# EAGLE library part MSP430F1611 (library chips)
IC MCU 16BIT 48KB FLASH
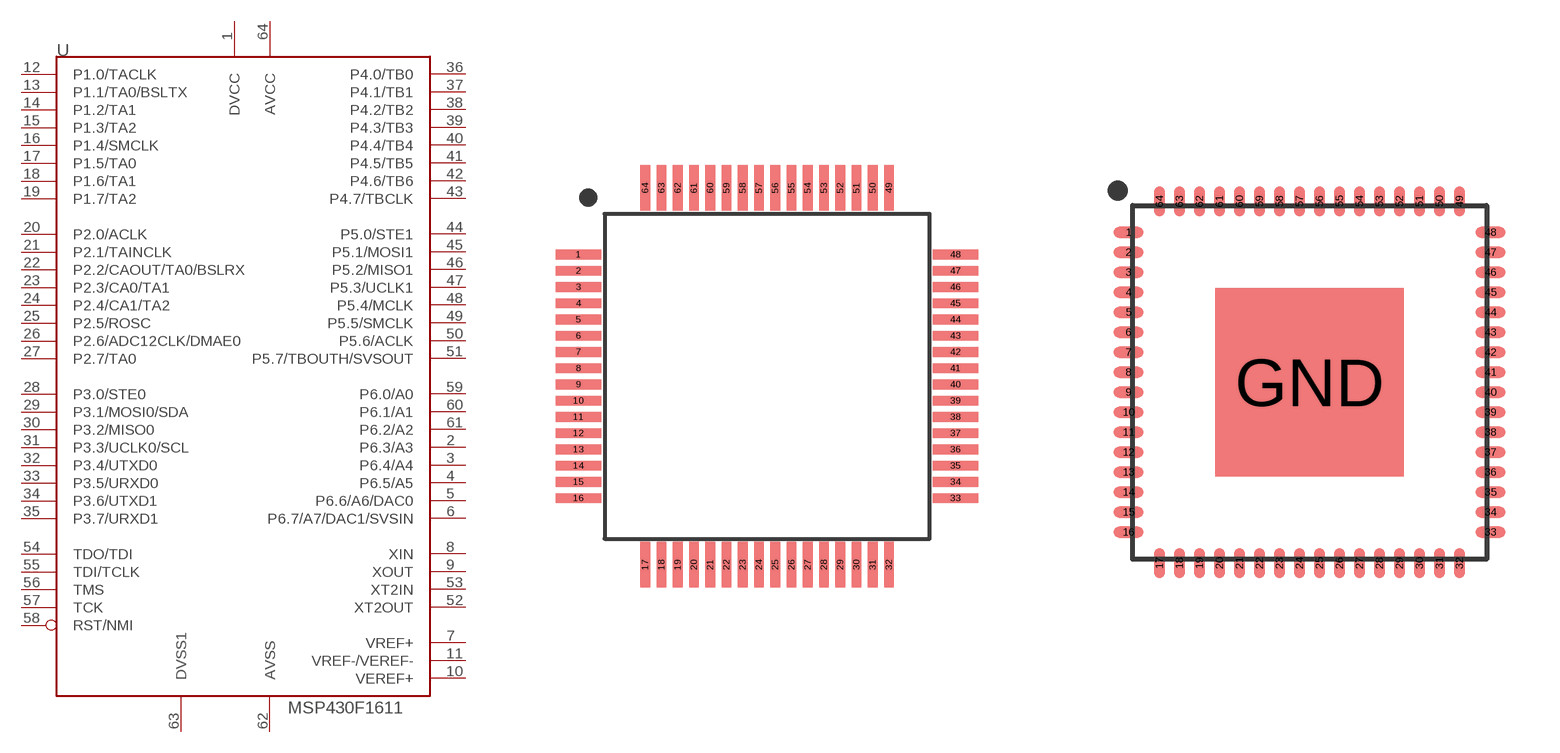
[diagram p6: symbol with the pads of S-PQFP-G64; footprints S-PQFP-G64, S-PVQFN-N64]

Designator prefix U

## MSP430F1611IPM (DIGIKEY: 296-26188-1-ND)  [S-PQFP-G64]
1  DVCC  pwr
2  P6.3/A3
3  P6.4/A4
4  P6.5/A5
5  P6.6/A6/DAC0
6  P6.7/A7/DAC1/SVSIN
7  VREF+
8  XIN
9  XOUT
10  VEREF+
11  VREF-/VEREF-
12  P1.0/TACLK
13  P1.1/TA0/BSLTX
14  P1.2/TA1
15  P1.3/TA2
16  P1.4/SMCLK
17  P1.5/TA0
18  P1.6/TA1
19  P1.7/TA2
20  P2.0/ACLK
21  P2.1/TAINCLK
22  P2.2/CAOUT/TA0/BSLRX
23  P2.3/CA0/TA1
24  P2.4/CA1/TA2
25  P2.5/ROSC
26  P2.6/ADC12CLK/DMAE0
27  P2.7/TA0
28  P3.0/STE0
29  P3.1/MOSI0/SDA
30  P3.2/MISO0
31  P3.3/UCLK0/SCL
32  P3.4/UTXD0
33  P3.5/URXD0
34  P3.6/UTXD1
35  P3.7/URXD1
36  P4.0/TB0
37  P4.1/TB1
38  P4.2/TB2
39  P4.3/TB3
40  P4.4/TB4
41  P4.5/TB5
42  P4.6/TB6
43  P4.7/TBCLK
44  P5.0/STE1
45  P5.1/MOSI1
46  P5.2/MISO1
47  P5.3/UCLK1
48  P5.4/MCLK
49  P5.5/SMCLK
50  P5.6/ACLK
51  P5.7/TBOUTH/SVSOUT
52  XT2OUT
53  XT2IN
54  TDO/TDI
55  TDI/TCLK
56  TMS
57  TCK
58  RST/NMI
59  P6.0/A0
60  P6.1/A1
61  P6.2/A2
62  AVSS  pwr
63  DVSS1  pwr
64  AVCC  pwr

## MSP430F1611IRTD (DIGIKEY: 296-18102-1-ND)  [S-PVQFN-N64]
1  DVCC  pwr
2  P6.3/A3
3  P6.4/A4
4  P6.5/A5
5  P6.6/A6/DAC0
6  P6.7/A7/DAC1/SVSIN
7  VREF+
8  XIN
9  XOUT
10  VEREF+
11  VREF-/VEREF-
12  P1.0/TACLK
13  P1.1/TA0/BSLTX
14  P1.2/TA1
15  P1.3/TA2
16  P1.4/SMCLK
17  P1.5/TA0
18  P1.6/TA1
19  P1.7/TA2
20  P2.0/ACLK
21  P2.1/TAINCLK
22  P2.2/CAOUT/TA0/BSLRX
23  P2.3/CA0/TA1
24  P2.4/CA1/TA2
25  P2.5/ROSC
26  P2.6/ADC12CLK/DMAE0
27  P2.7/TA0
28  P3.0/STE0
29  P3.1/MOSI0/SDA
30  P3.2/MISO0
31  P3.3/UCLK0/SCL
32  P3.4/UTXD0
33  P3.5/URXD0
34  P3.6/UTXD1
35  P3.7/URXD1
36  P4.0/TB0
37  P4.1/TB1
38  P4.2/TB2
39  P4.3/TB3
40  P4.4/TB4
41  P4.5/TB5
42  P4.6/TB6
43  P4.7/TBCLK
44  P5.0/STE1
45  P5.1/MOSI1
46  P5.2/MISO1
47  P5.3/UCLK1
48  P5.4/MCLK
49  P5.5/SMCLK
50  P5.6/ACLK
51  P5.7/TBOUTH/SVSOUT
52  XT2OUT
53  XT2IN
54  TDO/TDI
55  TDI/TCLK
56  TMS
57  TCK
58  RST/NMI
59  P6.0/A0
60  P6.1/A1
61  P6.2/A2
62  AVSS  pwr
63  DVSS1  pwr
64  AVCC  pwr
GND  DVSS1  pwr

## Footprint S-PQFP-G64 (pad centres in mm)
smd 1.4 x 0.3: 1 -5.8,3.75; 2 -5.8,3.25; 3 -5.8,2.75; 4 -5.8,2.25; 5 -5.8,1.75; 6 -5.8,1.25; 7 -5.8,0.75; 8 -5.8,0.25; 9 -5.8,-0.25; 10 -5.8,-0.75; 11 -5.8,-1.25; 12 -5.8,-1.75; 13 -5.8,-2.25; 14 -5.8,-2.75; 15 -5.8,-3.25; 16 -5.8,-3.75; 33 5.8,-3.75; 34 5.8,-3.25; 35 5.8,-2.75; 36 5.8,-2.25; 37 5.8,-1.75; 38 5.8,-1.25; 39 5.8,-0.75; 40 5.8,-0.25; 41 5.8,0.25; 42 5.8,0.75; 43 5.8,1.25; 44 5.8,1.75; 45 5.8,2.25; 46 5.8,2.75; 47 5.8,3.25; 48 5.8,3.75
smd 0.3 x 1.4: 17 -3.75,-5.8; 18 -3.25,-5.8; 19 -2.75,-5.8; 20 -2.25,-5.8; 21 -1.75,-5.8; 22 -1.25,-5.8; 23 -0.75,-5.8; 24 -0.25,-5.8; 25 0.25,-5.8; 26 0.75,-5.8; 27 1.25,-5.8; 28 1.75,-5.8; 29 2.25,-5.8; 30 2.75,-5.8; 31 3.25,-5.8; 32 3.75,-5.8; 49 3.75,5.8; 50 3.25,5.8; 51 2.75,5.8; 52 2.25,5.8; 53 1.75,5.8; 54 1.25,5.8; 55 0.75,5.8; 56 0.25,5.8; 57 -0.25,5.8; 58 -0.75,5.8; 59 -1.25,5.8; 60 -1.75,5.8; 61 -2.25,5.8; 62 -2.75,5.8; 63 -3.25,5.8; 64 -3.75,5.8

## Footprint S-PVQFN-N64 (pad centres in mm)
smd 0.75 x 0.28: 1 -4.525,3.75; 2 -4.525,3.25; 3 -4.525,2.75; 4 -4.525,2.25; 5 -4.525,1.75; 6 -4.525,1.25; 7 -4.525,0.75; 8 -4.525,0.25; 9 -4.525,-0.25; 10 -4.525,-0.75; 11 -4.525,-1.25; 12 -4.525,-1.75; 13 -4.525,-2.25; 14 -4.525,-2.75; 15 -4.525,-3.25; 16 -4.525,-3.75; 33 4.525,-3.75; 34 4.525,-3.25; 35 4.525,-2.75; 36 4.525,-2.25; 37 4.525,-1.75; 38 4.525,-1.25; 39 4.525,-0.75; 40 4.525,-0.25; 41 4.525,0.25; 42 4.525,0.75; 43 4.525,1.25; 44 4.525,1.75; 45 4.525,2.25; 46 4.525,2.75; 47 4.525,3.25; 48 4.525,3.75
smd 0.28 x 0.75: 17 -3.75,-4.525; 18 -3.25,-4.525; 19 -2.75,-4.525; 20 -2.25,-4.525; 21 -1.75,-4.525; 22 -1.25,-4.525; 23 -0.75,-4.525; 24 -0.25,-4.525; 25 0.25,-4.525; 26 0.75,-4.525; 27 1.25,-4.525; 28 1.75,-4.525; 29 2.25,-4.525; 30 2.75,-4.525; 31 3.25,-4.525; 32 3.75,-4.525; 49 3.75,4.525; 50 3.25,4.525; 51 2.75,4.525; 52 2.25,4.525; 53 1.75,4.525; 54 1.25,4.525; 55 0.75,4.525; 56 0.25,4.525; 57 -0.25,4.525; 58 -0.75,4.525; 59 -1.25,4.525; 60 -1.75,4.525; 61 -2.25,4.525; 62 -2.75,4.525; 63 -3.25,4.525; 64 -3.75,4.525
smd 4.7 x 4.7: GND 0,0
